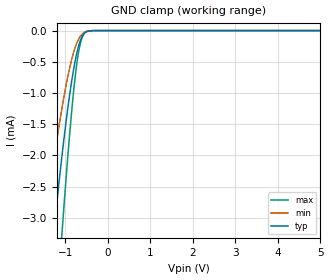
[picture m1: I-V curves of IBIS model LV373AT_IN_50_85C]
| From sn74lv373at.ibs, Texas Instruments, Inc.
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[Model]   LV373AT_IN_50_85C
Model_type  Input
Vinl=0.8
Vinh=2.0
| variable   typ   min   max
C_comp   4pF   NA   10pF
[Temperature Range]   40   100   -40
| Ambient temperature   25   85   -40
[Voltage range]   5   4.5   5.5
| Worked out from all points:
|   GND clamp passes 1 mA (typ) near -0.89 V on its own axis
[GND Clamp]
| LV373AT_IN_50
|   Voltage   I(typ)   I(min)   I(max)
-5V       -39.32mA   -26.34mA   -50.37mA
-1.54V    -5.154mA   -3.352mA   -7.998mA
-1.49V    -4.776mA   -3.1mA     -7.452mA
-1.28V    -3.276mA   -2.094mA   -5.225mA
-1.25V    -3.075mA   -1.959mA   -4.918mA
-1.08V    -2.002mA   -1.239mA   -3.244mA
-900mV    -1.03mA    -599.9uA   -1.659mA
-775mV    -504uA     -278.8uA   -770.4uA
-720mV    -327.9uA   -180.3uA   -474.1uA
-660mV    -182.1uA   -103.2uA   -240.1uA
-540mV    -34.71uA   -23.95uA   -34.46uA
5V        17.64nA    1.142nA    163.4nA
